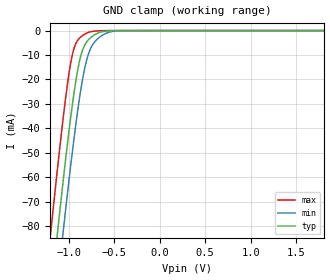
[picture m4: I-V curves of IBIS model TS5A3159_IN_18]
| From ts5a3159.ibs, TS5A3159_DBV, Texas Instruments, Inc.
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[Model]   TS5A3159_IN_18
Model_type  Input
Vinl=0.6
Vinh=1.5
| variable   typ   min   max
C_comp   1.96pF   1.60pF   2.33pF
[Temperature Range]   40   100   -40
| Ambient temperature   25   85   -40
[Voltage range]   1.8   1.65   1.95
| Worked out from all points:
|   GND clamp passes 1 mA (typ) near -0.68 V on its own axis
[GND Clamp]
| TS5A3159_IN_18
|   Voltage   I(typ)   I(min)   I(max)
-1.8V     -337mA     -357mA     -312.5mA
-1.2V     -110.8mA   -131.9mA   -84.38mA
-1.185V   -105.4mA   -126.5mA   -78.99mA
-1.12V    -82.43mA   -103.5mA   -56.15mA
-1.055V   -60.34mA   -81.11mA   -34.72mA
-965mV    -32.41mA   -51.87mA   -11.17mA
-890mV    -14.41mA   -30.36mA   -3.555mA
-825mV    -6.156mA   -15.91mA   -1.509mA
-775mV    -3.522mA   -8.911mA   -658.3uA
-715mV    -1.758mA   -4.71mA    -243.8uA
-510mV    -44.15uA   -301.4uA   -925nA
1.8V      32.58pA    2.059nA    21.61pA
